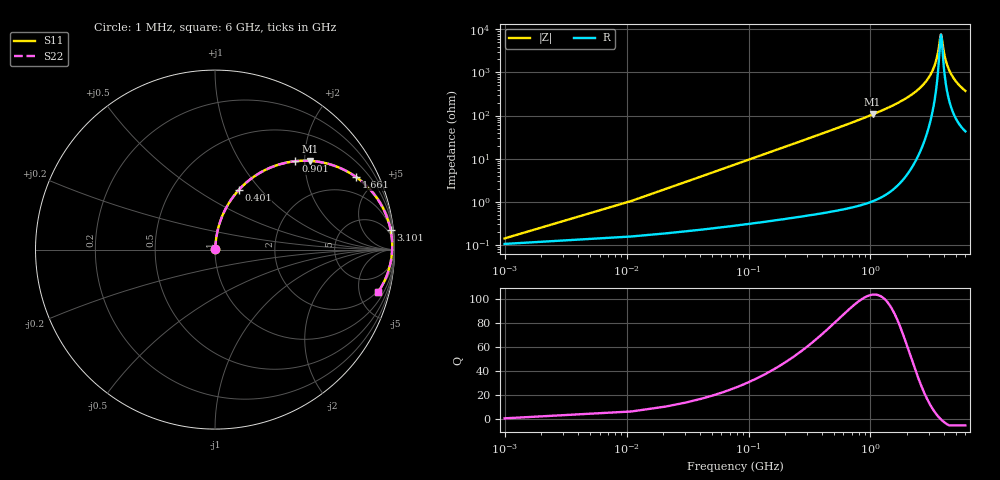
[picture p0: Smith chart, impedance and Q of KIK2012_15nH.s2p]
!version-2
!date-01.2022
!Series
# MHz S RI R 50
!Freq ReS11 ImS11 ReS21 ImS21 ReS12 ImS12 ReS22 ImS22
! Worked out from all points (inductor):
!   601 points, 1 MHz to 6 GHz, reference 50 ohm
!   read as one part in series: L = 15 nH near 31 MHz
!   highest Q = 104 at 1.041 GHz (marker M1), where L = 16.2 nH
!   self-resonance near 3.786 GHz
!   S11 on the Smith chart (normalised r, x): 1 MHz: 1.00, +0.00; 401 MHz: 1.01, +0.76; 901 MHz: 1.02, +1.80; 1.661 GHz: 1.05, +3.88; 3.101 GHz: 2, +18; 6 GHz: 1.86, -7.42
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1  0.00105 0.00094  0.9989 -0.00094  0.9989 -0.00094  0.00105 0.00094
41  0.00373 0.0384  0.9963 -0.0384  0.9963 -0.0384  0.00373 0.0384
61  0.00583 0.057  0.9942 -0.057  0.9942 -0.057  0.00583 0.057
91  0.0102 0.0847  0.9898 -0.0847  0.9898 -0.0847  0.0102 0.0847
141  0.0207 0.1299  0.9793 -0.1299  0.9793 -0.1299  0.0207 0.1299
211  0.0419 0.1904  0.9581 -0.1904  0.9581 -0.1904  0.0419 0.1904
401  0.131 0.3304  0.869 -0.3304  0.869 -0.3304  0.131 0.3304
901  0.4482 0.4924  0.5518 -0.4924  0.5518 -0.4924  0.4482 0.4924
1001  0.5071 0.4951  0.4929 -0.4951  0.4929 -0.4951  0.5071 0.4951
1041  0.5295 0.4943  0.4705 -0.4943  0.4705 -0.4943  0.5295 0.4943
1661  0.7871 0.4034  0.2129 -0.4034  0.2129 -0.4034  0.7871 0.4034
2001  0.8686 0.3297  0.1314 -0.3297  0.1314 -0.3297  0.8686 0.3297
3001  0.9745 0.1268  0.0255 -0.1268  0.0255 -0.1268  0.9745 0.1268
3101  0.9784 0.109  0.0216 -0.109  0.0216 -0.109  0.9784 0.109
3471  0.9865 0.0475  0.0135 -0.0475  0.0135 -0.0475  0.9865 0.0475
3771  0.9871 0.00223  0.0129 -0.00223  0.0129 -0.00223  0.9871 0.00223
3831  0.9867 -0.00637  0.0133 0.00637  0.0133 0.00637  0.9867 -0.00637
4001  0.9848 -0.0299  0.0152 0.0299  0.0152 0.0299  0.9848 -0.0299
4161  0.9821 -0.0511  0.0179 0.0511  0.0179 0.0511  0.9821 -0.0511
4381  0.977 -0.0786  0.023 0.0786  0.023 0.0786  0.977 -0.0786
5001  0.956 -0.1473  0.044 0.1473  0.044 0.1473  0.956 -0.1473
6000  0.9096 -0.2347  0.0904 0.2347  0.0904 0.2347  0.9096 -0.2347
